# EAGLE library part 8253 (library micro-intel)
MICROCOMPUTER/PERIPHERAL DEVICE
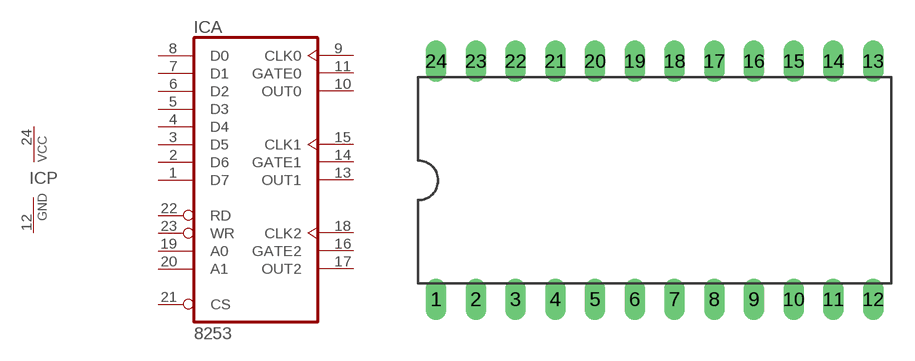
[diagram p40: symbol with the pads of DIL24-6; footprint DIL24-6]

Designator prefix IC; gates A=8253 P=PWRN

## 8253 (OC_FARNELL: unknown; OC_NEWARK: unknown)  [DIL24-6]
1  A:D7
2  A:D6
3  A:D5
4  A:D4
5  A:D3
6  A:D2
7  A:D1
8  A:D0
9  A:CLK0  in
10  A:OUT0  out
11  A:GATE0  in
12  P:GND  pwr
13  A:OUT1  out
14  A:GATE1  in
15  A:CLK1  in
16  A:GATE2  in
17  A:OUT2  out
18  A:CLK2  in
19  A:A0  in
20  A:A1  in
21  A:CS  in
22  A:RD  in
23  A:WR  in
24  P:VCC  pwr

## Footprint DIL24-6 (pad centres in mm)
Dual In Line Package 0.6 inch
drill 0.813 long: 1 -13.97,-7.62; 2 -11.43,-7.62; 3 -8.89,-7.62; 4 -6.35,-7.62; 5 -3.81,-7.62; 6 -1.27,-7.62; 7 1.27,-7.62; 8 3.81,-7.62; 9 6.35,-7.62; 10 8.89,-7.62; 11 11.43,-7.62; 12 13.97,-7.62; 13 13.97,7.62; 14 11.43,7.62; 15 8.89,7.62; 16 6.35,7.62; 17 3.81,7.62; 18 1.27,7.62; 19 -1.27,7.62; 20 -3.81,7.62; 21 -6.35,7.62; 22 -8.89,7.62; 23 -11.43,7.62; 24 -13.97,7.62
